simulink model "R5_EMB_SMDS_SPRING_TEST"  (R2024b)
settings: Solver=ode5  StartTime=0.0  StopTime=S  FixedStep=T  RelTol=1e-3  EnableMultiTasking=on
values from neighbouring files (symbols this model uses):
  Kt = 0.0273    [R5_EMB_SMDS_SPRING_TEST_script.m]
  r_act = 0.0105    [R5_EMB_SMDS_SPRING_TEST_script.m]
  T = 0.002    [R5_EMB_SMDS_SPRING_TEST_script.m]
undefined symbols (not defined in the file or in its folder): Serial_Port, Standard_Devices
libraries: easyio x6, simulink x2

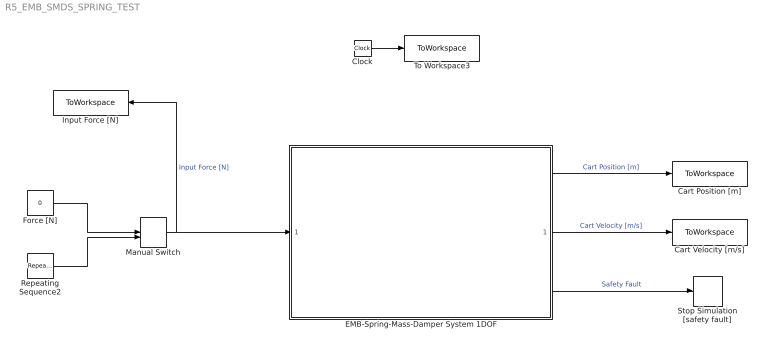
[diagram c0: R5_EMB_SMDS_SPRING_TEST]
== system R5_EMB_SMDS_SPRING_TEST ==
  Cart Position [m] : ToWorkspace  VariableName=cart_position  SampleTime=-1
  Cart Velocity [m/s] : ToWorkspace  VariableName=cart_velocity  SampleTime=-1
  Clock : Clock
  EMB-Spring-Mass-Damper System 1DOF : Subsystem
  Force [N] : Constant  Value=0
  Input Force [N] : ToWorkspace  VariableName=f_input  SampleTime=-1
  Manual Switch : ManualSwitch  CurrentSetting=0
  Repeating Sequence2 : simulink/Sources/Repeating Sequence  rep_seq_t=[0 1 2 3 4 5 6]  rep_seq_y=[0 2 4 6 8 10 0]
  Stop Simulation [safety fault] : Stop
  To Workspace3 : ToWorkspace  VariableName=rt_time  SampleTime=-1
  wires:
  Clock/1 -> To Workspace3/1
  EMB-Spring-Mass-Damper System 1DOF/1(Out1) -> Cart Position [m]/1  "Cart Position [m]"
  EMB-Spring-Mass-Damper System 1DOF/3(Out3) -> Stop Simulation [safety fault]/1  "Safety Fault"
  Manual Switch/1 -> Input Force [N]/1, EMB-Spring-Mass-Damper System 1DOF/1(In1)  "Input Force [N]"
  Repeating Sequence2/1 -> Manual Switch/2
  Force [N]/1 -> Manual Switch/1
  EMB-Spring-Mass-Damper System 1DOF/2(Out2) -> Cart Velocity [m/s]/1  "Cart Velocity [m/s]"

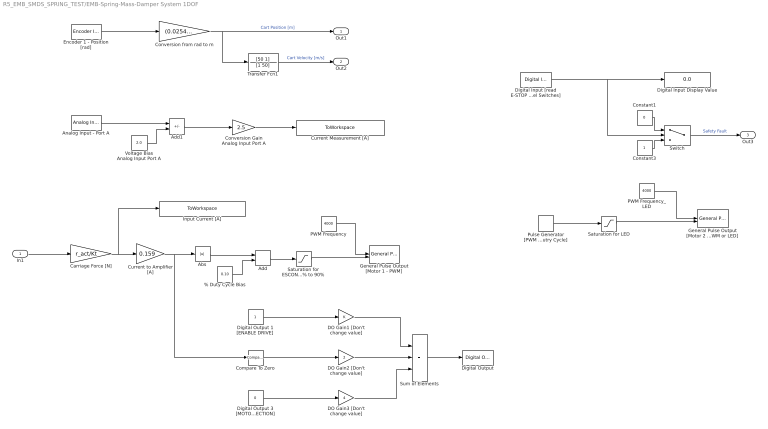
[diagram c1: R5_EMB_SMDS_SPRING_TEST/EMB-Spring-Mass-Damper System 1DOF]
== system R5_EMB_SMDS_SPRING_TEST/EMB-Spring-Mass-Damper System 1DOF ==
  In1 : Inport
  % Duty Cycle Bias : Constant  Value=0.10
  Abs : Abs
  Add : Sum
  Add1 : Sum  Inputs=+-
  Analog Input - Port A : easyio/Analog Input  SampleTime=T  MaxMissedTicks=10  ShowMissedTicks=0  YieldWhenWaiting=0  DrvName=Standard_Devices/Serial_Port  DrvAddress=6  DrvOptions=[460800 8 0 0 0 0 0 0]  PacketSize=8  DataTypes='double'  ShowReady=0  ShowError=0  PacketID=1  ByteOrder=1  ShowTimestamp=0  CfgPrm=A6  PrmCfg=unipolar  ResVar=0  VarRes=0
  Carriage Force [N] : Gain  Gain=r_act/Kt
  Compare To Zero : simulink/Logic and Bit Operations/Compare To Zero  relop=>=  OutDataTypeStr=boolean
  Constant1 : Constant  Value=0
  Constant3 : Constant
  Conversion Gain Analog Input Port A : Gain  Gain=2.5
  Conversion from rad to m : Gain  Gain=(0.0254)/(2*pi)
  Current Measurement [A] : ToWorkspace  VariableName=i_measure  SampleTime=-1
  Current to Amplifier [A] : Gain  Gain=0.159
  DO Gain1 [Don't change value] : Gain
  DO Gain2 [Don't change value] : Gain  Gain=2
  DO Gain3 [Don't change value] : Gain  Gain=4
  Digital Input Display Value : Display
  Digital Input [read E-STOP and End of Travel Switches] : easyio/Digital Input  SampleTime=T  MaxMissedTicks=10  ShowMissedTicks=0  YieldWhenWaiting=0  DrvName=Standard_Devices/Serial_Port  DrvAddress=6  DrvOptions=[460800 8 0 0 0 0 0 0]  PacketSize=8  DataTypes='double'  ShowReady=0  ShowError=0  PacketID=1  ByteOrder=1  ShowTimestamp=0  CfgPrm=D0  PrmCfg=18  ResVar=0  VarRes=0  d7=off  d6=off  d5=off  d4=on  d3=on  d2=off  d1=off  d0=off
  Digital Output : easyio/Digital Output  SampleTime=T  MaxMissedTicks=10  ShowMissedTicks=0  YieldWhenWaiting=0  DrvName=Standard_Devices/Serial_Port  DrvAddress=6  DrvOptions=[460800 8 0 0 0 0 0 0]  PacketSize=8  DataTypes='double'  ShowReady=0  ShowError=0  PacketID=1  ByteOrder=1  InitialValue=0  FinalValue=0  CfgPrm=G0  PrmCfg=F8  ResVar=0  VarRes=0  d7=off  d6=off  d5=off  d4=off  d3=off  d2=on  d1=on  d0=on
  Digital Output 1 [ENABLE DRIVE] : Constant
  Digital Output 3 [MOTOR 2 DIRECTION] : Constant  Value=0
  Encoder 1 - Position [rad] : easyio/Encoder Input  SampleTime=T  MaxMissedTicks=10  ShowMissedTicks=0  YieldWhenWaiting=0  DrvName=Standard_Devices/Serial_Port  DrvAddress=6  DrvOptions=[460800 8 0 0 0 0 0 0]  PacketSize=8  DataTypes='double'  ShowReady=0  ShowError=0  PacketID=1  ByteOrder=1  ShowTimestamp=0  CfgPrm=E0  PrmCfg=position  ResVar=0  VarRes=2000
  General Pulse Output [Motor 1 - PWM] : easyio/General Pulse Output  SampleTime=T  MaxMissedTicks=10  ShowMissedTicks=0  YieldWhenWaiting=0  DrvName=Standard_Devices/Serial_Port  DrvAddress=6  DrvOptions=[460800 8 0 0 0 0 0 0]  PacketSize=16  DataTypes={'double','double'}  ShowReady=0  ShowError=0  PacketID=1  ByteOrder=1  InitialValue=[0 0]  FinalValue=[0 0]  CfgPrm=N0  PrmCfg=frequency and duty  ResVar=449.8360 Hz - 115156.25 Hz  VarRes=64
  General Pulse Output [Motor 2 - PWM or LED] : easyio/General Pulse Output  SampleTime=T  MaxMissedTicks=10  ShowMissedTicks=0  YieldWhenWaiting=0  DrvName=Standard_Devices/Serial_Port  DrvAddress=6  DrvOptions=[460800 8 0 0 0 0 0 0]  PacketSize=16  DataTypes={'double','double'}  ShowReady=0  ShowError=0  PacketID=1  ByteOrder=1  InitialValue=[0 0]  FinalValue=[0 0]  CfgPrm=N1  PrmCfg=frequency and duty  ResVar=449.8360 Hz - 115156.25 Hz  VarRes=64
  Input Current [A] : ToWorkspace  VariableName=i_input  SampleTime=-1
  PWM Frequency : Constant  Value=4000
  PWM Frequency_LED : Constant  Value=4000
  Pulse Generator [PWM % Dutry Cycle] : DiscretePulseGenerator  PulseType=Time based  Period=0.4  PulseWidth=50
  Saturation for ESCON 10% to 90% : Saturate  UpperLimit=0.9  LowerLimit=0.1
  Saturation for LED : Saturate  UpperLimit=1  LowerLimit=0
  Sum of Elements : Sum  Inputs=+++
  Switch : Switch  Threshold=24
  Transfer Fcn1 : TransferFcn  Numerator=[50 1]  Denominator=[1 50]
  Voltage Bias Analog Input Port A : Constant  Value=2.0
  Out1 : Outport
  Out2 : Outport  Port=2
  Out3 : Outport  Port=3
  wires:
  Switch/1 -> Out3/1  "Safety Fault"
  % Duty Cycle Bias/1 -> Add/2
  Conversion Gain Analog Input Port A/1 -> Current Measurement [A]/1
  Add1/1 -> Conversion Gain Analog Input Port A/1
  Constant1/1 -> Switch/1
  Current to Amplifier [A]/1 -> Abs/1, Compare To Zero/1
  Saturation for ESCON 10% to 90%/1 -> General Pulse Output [Motor 1 - PWM]/2
  Voltage Bias Analog Input Port A/1 -> Add1/2
  DO Gain2 [Don't change value]/1 -> Sum of Elements/2
  Analog Input - Port A/1 -> Add1/1
  PWM Frequency/1 -> General Pulse Output [Motor 1 - PWM]/1
  Conversion from rad to m/1 -> Out1/1, Transfer Fcn1/1  "Cart Position [m]"
  DO Gain1 [Don't change value]/1 -> Sum of Elements/1
  Digital Output 1 [ENABLE DRIVE]/1 -> DO Gain1 [Don't change value]/1
  Saturation for LED/1 -> General Pulse Output [Motor 2 - PWM or LED]/2
  Digital Input [read E-STOP and End of Travel Switches]/1 -> Switch/2, Digital Input Display Value/1
  PWM Frequency_LED/1 -> General Pulse Output [Motor 2 - PWM or LED]/1
  Carriage Force [N]/1 -> Input Current [A]/1, Current to Amplifier [A]/1
  Pulse Generator [PWM % Dutry Cycle]/1 -> Saturation for LED/1
  Encoder 1 - Position [rad]/1 -> Conversion from rad to m/1
  Sum of Elements/1 -> Digital Output/1
  Add/1 -> Saturation for ESCON 10% to 90%/1
  Constant3/1 -> Switch/3
  Compare To Zero/1 -> DO Gain2 [Don't change value]/1
  Abs/1 -> Add/1
  In1/1 -> Carriage Force [N]/1
  Digital Output 3 [MOTOR 2 DIRECTION]/1 -> DO Gain3 [Don't change value]/1
  DO Gain3 [Don't change value]/1 -> Sum of Elements/3
  Transfer Fcn1/1 -> Out2/1  "Cart Velocity [m/s]"
